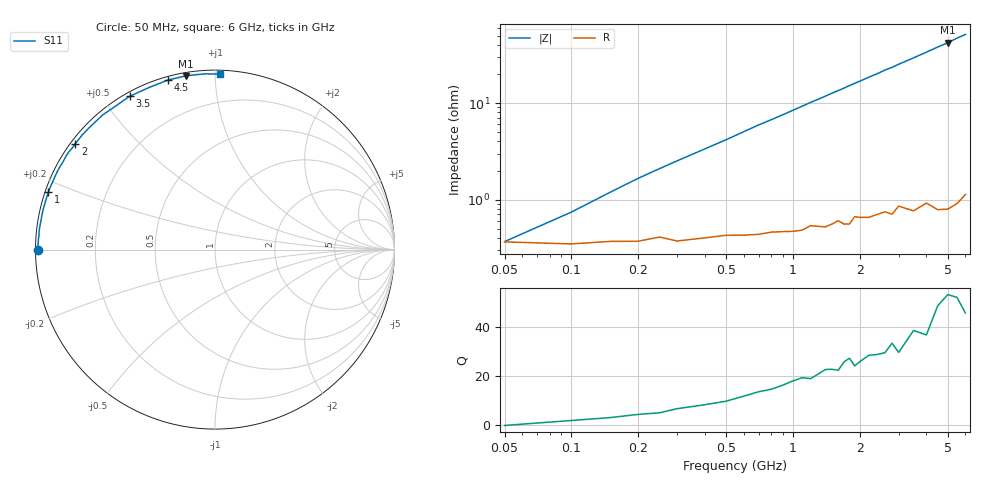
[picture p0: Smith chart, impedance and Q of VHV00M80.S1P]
! Infineon Technologies  Discrete & RF Semiconductors
! BB 814
! Si Tuning Diode in SOT23
! VR =
! S-Parameters:  July  1999
# GHz  S  MA  R  50
!  f  S11
! GHz  MAG  ANG
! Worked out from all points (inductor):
!   34 points, 50 MHz to 6 GHz, reference 50 ohm
!   read as one part to ground: L = 1.29 nH near 150 MHz
!   highest Q = 51.9 at 5 GHz (marker M1), where L = 1.34 nH
!   S11 on the Smith chart (normalised r, x): 50 MHz: 0.01, -0.00; 1 GHz: 0.01, +0.17; 2 GHz: 0.01, +0.34; 3.5 GHz: 0.02, +0.59; 4.5 GHz: 0.02, +0.76; 6 GHz: 0.02, +1.03
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0.05  0.9855 -179.9
0.1  0.9862 178.5
0.2  0.9853 176.3
0.25  0.9838 175.3
0.3  0.9853 174.3
0.5  0.9832 170.5
0.7  0.983 166.5
0.8  0.9821 164.7
1  0.982 160.9
1.2  0.9796 157.1
1.4  0.9805 153.5
1.5  0.9793 151.6
1.6  0.9778 149.9
1.7  0.9796 148.1
1.8  0.9798 146.2
1.9  0.9761 144.5
2  0.9768 142.8
2.2  0.9773 139.3
2.4  0.9761 136.1
2.6  0.9753 132.6
2.8  0.9772 129.7
3  0.9731 126.4
3.5  0.9776 119.1
4  0.975 112.0
4.5  0.9803 105.4
5  0.9816 99.6
5.5  0.9809 93.4
6  0.9783 88.4
